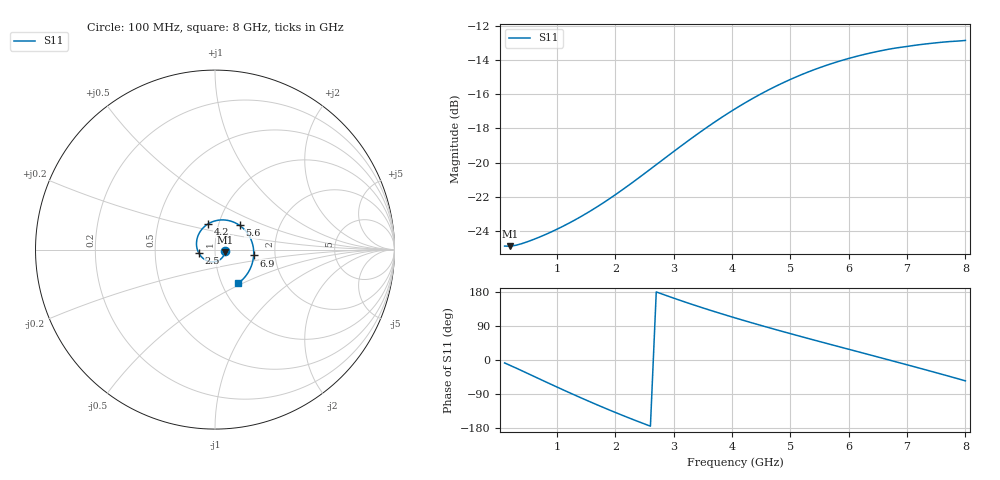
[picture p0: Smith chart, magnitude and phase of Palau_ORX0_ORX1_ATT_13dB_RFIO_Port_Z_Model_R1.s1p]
! Created Fri Oct  9 14:28:24 2020
! Palau ORX0/ORX1 RFIO Port Impedance Model.
! Attenuation  : 13 dB.
! Revision		: R1.
! Impedance Mode 	: Balanced Differential-Mode.
! Impedance Format 	: Series Equivalent Differential Impedance (SEDZ).
# hz S ma R 100
! 1 Port Network Data from SP1.SP block
! freq  magS11  angS11
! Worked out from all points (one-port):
!   80 points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, 100 MHz to 8 GHz, reference 100 ohm
!   lowest |S11| = -24.9 dB at 200 MHz (marker M1), VSWR 1.12, Z = 112 - j3.21 ohm
!   |S11| at or under -10 dB: start of sweep to end of sweep
!   S11 on the Smith chart (normalised r, x): 100 MHz: 1.12, -0.02; 2.5 GHz: 0.83, -0.03; 4.2 GHz: 0.89, +0.26; 5.6 GHz: 1.26, +0.35; 6.9 GHz: 1.54, -0.11; 8 GHz: 1.20, -0.47
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1e8  0.05688 -7.8
2e8  0.05685 -14.6
6e8  0.05952 -43.0
1.1e9  0.06502 -78.5
1.4e9  0.06929 -99.2
1.6e9  0.0726 -112.6
1.8e9  0.07633 -125.7
2.1e9  0.08274 -144.7
2.5e9  0.09286 -168.8
2.8e9  0.1015 174.1
3.1e9  0.111 157.9
3.3e9  0.1176 147.5
3.6e9  0.1279 132.5
4.1e9  0.1454 108.9
4.2e9  0.1488 104.4
4.5e9  0.1591 91.0
4.7e9  0.1657 82.3
5.1e9  0.1783 65.4
5.3e9  0.1841 57.0
5.6e9  0.1923 44.6
5.8e9  0.1973 36.5
6.1e9  0.2041 24.2
6.5e9  0.2118 7.9
6.9e9  0.2178 -8.6
7.1e9  0.2202 -16.8
7.5e9  0.2244 -33.6
7.7e9  0.2261 -42.1
8e9  0.228 -55.0
